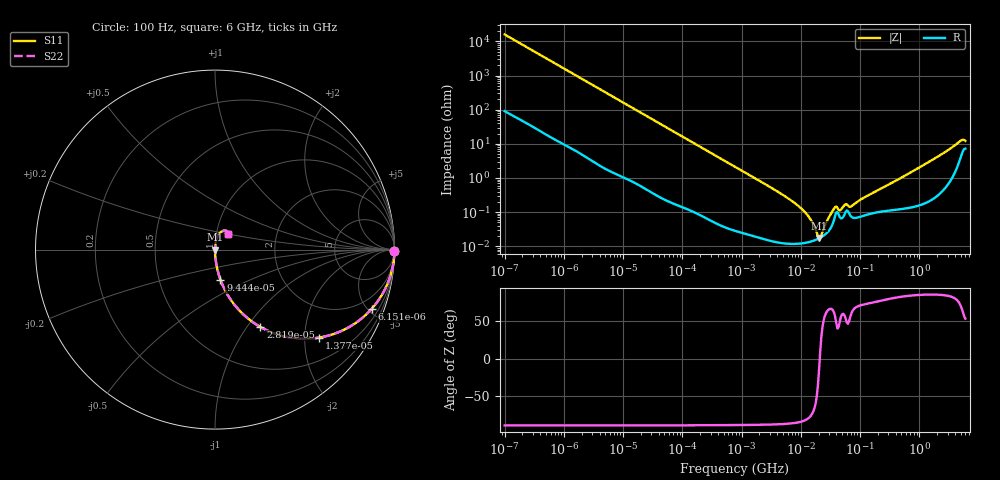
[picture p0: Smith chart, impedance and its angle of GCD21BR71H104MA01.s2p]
!Murata Part Number: GCD21BR71H104MA01
!These Parameters are Measured in Series Mode Connection
!Data Generated on Jan 08, 2026
!  o--ll--o
!Port1  Port2
!  o------o
!Operation Temp=25[degC], DC Bias Voltage=0[V]
!Freq. Start=100[Hz] Stop=6[GHz] 401[Steps]
# Hz S RI R 50
!Freq.(Hz) S11(Real) S11(Imag) S21(Real) S21(Imag) S12(Real) S12(Imag) S22(Real) S22(Imag)
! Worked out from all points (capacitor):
!   401 points, 100 Hz to 6 GHz, reference 50 ohm
!   read as one part in series: C = 99.5 nF near 109 Hz
!   lowest |Z| = 17.5 mohm at 20.35 MHz (marker M1)
!   series resonance near 20.89 MHz, so ESL is about 580 pH
!   S11 on the Smith chart (normalised r, x): 100 Hz: open; 6.151 kHz: 1.03, -5.27; 13.77 kHz: 1.02, -2.36; 28.19 kHz: 1.01, -1.16; 94.44 kHz: 1.00, -0.35; 6 GHz: 1.14, +0.20
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100  0.9999 -0.00626  7.49e-05 0.00626  7.49e-05 0.00626  0.9999 -0.00626
2008  0.9841 -0.1222  0.0159 0.1222  0.0159 0.1222  0.9841 -0.1222
6151  0.8727 -0.3304  0.1273 0.3304  0.1273 0.3304  0.8727 -0.3304
13772  0.5819 -0.4898  0.4181 0.4898  0.4181 0.4898  0.5819 -0.4898
28191  0.2525 -0.431  0.7475 0.431  0.7475 0.431  0.2525 -0.431
40335  0.1428 -0.3464  0.8572 0.3464  0.8572 0.3464  0.1428 -0.3464
94437  0.0306 -0.1681  0.9694 0.1681  0.9694 0.1681  0.0306 -0.1681
774597  0.000738 -0.0214  0.9993 0.0214  0.9993 0.0214  0.000738 -0.0214
6948629  0.000121 -0.00216  0.9999 0.00216  0.9999 0.00216  0.000121 -0.00216
1.137099e7  0.000125 -0.00105  0.9999 0.00105  0.9999 0.00105  0.000125 -0.00105
1.555665e7  0.000141 -0.000488  0.9999 0.000488  0.9999 0.000488  0.000141 -0.000488
2.035112e7  0.00017 -4.28e-05  0.9998 4.28e-05  0.9998 4.28e-05  0.00017 -4.28e-05
2.225763e7  0.000185 0.000107  0.9998 -0.000107  0.9998 -0.000107  0.000185 0.000107
2.911731e7  0.000272 0.000596  0.9997 -0.000596  0.9997 -0.000596  0.000272 0.000596
3.80911e7  0.000793 0.00116  0.9992 -0.00116  0.9992 -0.00116  0.000793 0.00116
4.556224e7  0.00071 0.000852  0.9993 -0.000852  0.9993 -0.000852  0.00071 0.000852
5.699437e7  0.000999 0.00137  0.999 -0.00137  0.999 -0.00137  0.000999 0.00137
7.129496e7  0.000731 0.00129  0.9993 -0.00129  0.9993 -0.00129  0.000731 0.00129
3.124326e8  0.00115 0.00642  0.9989 -0.00642  0.9989 -0.00642  0.00115 0.00642
1.873145e9  0.00415 0.038  0.9959 -0.038  0.9959 -0.038  0.00415 0.038
4.796499e9  0.0427 0.1038  0.9573 -0.1038  0.9573 -0.1038  0.0427 0.1038
6e9  0.0751 0.0848  0.9249 -0.0848  0.9249 -0.0848  0.0751 0.0848
